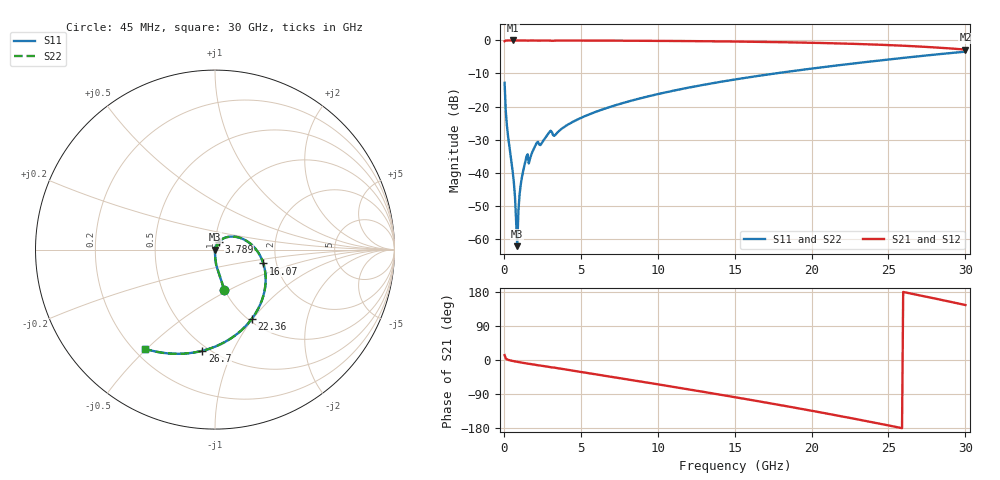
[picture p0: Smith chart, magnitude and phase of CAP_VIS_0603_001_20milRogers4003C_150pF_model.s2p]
! S-parameter model data by Modelithics Inc.  support@modelithics.com  813-866-6335  Tampa FL USA
! S-Parameter data specifications:
! Substrate: 20-mil Rogers 4003C, substrate thickness, H=0.508mm, Dielectric constant, Er=3.75
! PCB Mounting Pad Footprint: Pad width, PadW=0.90mm , Pad length, PadL=1.00mm , Pad gap, PadG (edge-to-edge)=1.00mm , Reference planes=3.0mm apart
! Created Wed Nov 18 13:32:20 2015
# hz S ma R 50
! 2 Port Network Data from SP1.SP block
! freq  magS11  angS11  magS21  angS21  magS12  angS12  magS22  angS22
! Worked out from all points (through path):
!   401 points, 45 MHz to 30 GHz, reference 50 ohm
!   highest |S21| = -0.01 dB at 569.2 MHz (marker M1); lowest = -2.8 dB at 30 GHz (marker M2)
!   group delay of S21, straight-line fit = 19.7 ps
!   lowest |S11| = -62.3 dB at 868.8 MHz (marker M3), VSWR 1.00, Z = 50.1 + j0.0438 ohm
!   |S11| at or under -10 dB: start of sweep to 17.63 GHz
!   |S22| runs from -62.3 to -3.4 dB; largest |S21 - S12| = 0
!   S11 on the Smith chart (normalised r, x): 45 MHz: 1.00, -0.47; 3.789 GHz: 1.04, +0.09; 16.07 GHz: 1.71, -0.29; 22.36 GHz: 1.03, -0.99; 26.7 GHz: 0.46, -0.77; 30 GHz: 0.24, -0.49
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4.5e7  0.2284 -77.0  0.9734 13.0  0.9734 13.0  0.2284 -77.0
2.696625e8  0.03535 -88.9  0.999 0.5  0.999 0.5  0.03535 -88.9
5.692125e8  0.01039 -89.9  0.9994 -2.6  0.9994 -2.6  0.01039 -89.9
7.189875e8  0.004336 -86.6  0.9994 -3.7  0.9994 -3.7  0.004336 -86.6
8.687625e8  0.0007696 34.6  0.9993 -4.8  0.9993 -4.8  0.0007696 34.6
1.018538e9  0.004656 76.0  0.9992 -5.9  0.9992 -5.9  0.004656 76.0
1.168312e9  0.008453 78.0  0.9991 -7.0  0.9991 -7.0  0.008453 78.0
1.392975e9  0.01461 76.4  0.9985 -8.5  0.9985 -8.5  0.01461 76.4
1.767412e9  0.01833 74.4  0.9982 -10.8  0.9982 -10.8  0.01833 74.4
2.066962e9  0.02636 71.5  0.9969 -12.9  0.9969 -12.9  0.02636 71.5
2.890725e9  0.03905 66.5  0.9954 -18.2  0.9954 -18.2  0.03905 66.5
3.34005e9  0.0372 61.9  0.9942 -20.6  0.9942 -20.6  0.0372 61.9
3.789375e9  0.04669 63.9  0.9966 -23.6  0.9966 -23.6  0.04669 63.9
5.062462e9  0.06814 56.8  0.9956 -31.9  0.9956 -31.9  0.06814 56.8
1.007992e10  0.1555 24.6  0.9849 -64.6  0.9849 -64.6  0.1555 24.6
1.50225e10  0.2567 -8.7  0.9626 -98.1  0.9626 -98.1  0.2567 -8.7
1.607092e10  0.2801 -16.0  0.9558 -105.5  0.9558 -105.5  0.2801 -16.0
2.003996e10  0.3758 -44.6  0.9216 -134.2  0.9216 -134.2  0.3758 -44.6
2.236148e10  0.4378 -62.2  0.8933 -151.8  0.8933 -151.8  0.4378 -62.2
2.505742e10  0.5164 -83.5  0.8497 -173.1  0.8497 -173.1  0.5164 -83.5
2.670495e10  0.568 -97.1  0.8157 173.3  0.8157 173.3  0.568 -97.1
3e10  0.6765 -125.2  0.7276 145.2  0.7276 145.2  0.6765 -125.2
